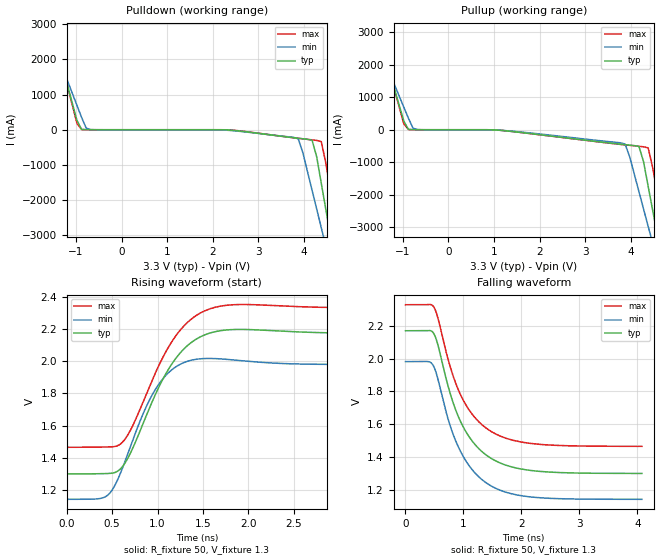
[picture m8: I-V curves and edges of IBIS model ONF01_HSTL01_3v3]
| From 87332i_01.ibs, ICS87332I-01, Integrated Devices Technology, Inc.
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[Model] ONF01_HSTL01_3v3
Model_type  Output_ECL
Polarity   Non-Inverting
Vmeas = 1.56
Rref = 50
Cref = 0
Vref = 1.3
|   typ   min   max
C_comp   4pF   3.6pF   4.4pF
|   typ   min   max
[Temperature Range]   25   -40   85
|   typ   min   max
[Voltage range]   3.3V   3.135V   3.465V
|   typ   min   max
[Pullup Reference]   3.3V   3.135V   3.465V
|   typ   min   max
[Pulldown Reference]   3.3V   3.135V   3.465V
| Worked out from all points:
|   rising waveform, R_fixture 50, V_fixture 1.3: 20-80 % time 436ps typ, 369ps min, 442ps max; typ from 1.3 V to 2.17 V
|   falling waveform, R_fixture 50, V_fixture 1.3: 20-80 % time 585ps typ, 578ps min, 582ps max; typ from 2.17 V to 1.3 V
| Open source, no load
|  Voltage   I(typ)   I(min)   I(max)
[Pulldown]
-3.3V     11.43A     8.569A     12.06A
-1.583V   3.173A     2.741A     3.273A
-1.482V   2.688A     2.399A     2.757A
-976.5mV  265.3mA    691.7mA    179.8mA
-875.5mV  9.277mA    351.3mA    5.817mA
-673.5mV  497.4uA    4.407mA    311.2uA
3.872V    -242.5mA   -258.2mA   -243.1mA
4.176V    -296.5mA   -1.72A     -288.3mA
4.378V    -1.523A    -2.788A    -338.2mA
4.58V     -3.033A    -3.855A    -1.761A
4.782V    -4.544A    -4.922A    -3.367A
6.6V      -18.28A    -14.6A     -17.98A
|  Voltage   I(typ)   I(min)   I(max)
[Pullup]
-3.3V     11.43A     8.569A     12.06A
-1.785V   4.144A     3.426A     4.306A
-1.583V   3.173A     2.741A     3.273A
-976.5mV  265.3mA    691.7mA    179.8mA
-875.5mV  9.277mA    351.3mA    5.817mA
-673.5mV  497.4uA    4.407mA    311.2uA
3.872V    -459.3mA   -442.5mA   -466.1mA
4.176V    -512mA     -1.904A    -509.8mA
4.378V    -1.738A    -2.972A    -558.7mA
4.58V     -3.247A    -4.039A    -1.98A
4.782V    -4.756A    -5.105A    -3.585A
6.6V      -18.37A    -14.72A    -18.06A
[Ramp]
|   typ   min   max
dV/dt_r   0.716/0.687n   0.698/0.591n   0.708/0.691n
dV/dt_f   0.696/0.94n   0.671/0.923n   0.691/0.935n
R_load =   50.0000
[Rising Waveform]
R_fixture = 50
V_fixture = 1.3   | VCC_typ - 2V
V_fixture_max = 1.465   | VCC_max - 2V
V_fixture_min = 1.135   | VCC_min - 2V
C_fixture = 0.0p
| Time   typ   min   max
0s        1.3V       1.142V     1.465V
427.6ps   1.302V     1.159V     1.467V
612.1ps   1.344V     1.334V     1.496V
731ps     1.465V     1.516V     1.605V
960.6ps   1.774V     1.81V      1.907V
1.121ns   1.95V      1.928V     2.087V
1.301ns   2.081V     1.993V     2.224V
1.522ns   2.163V     2.015V     2.312V
1.805ns   2.194V     2.008V     2.348V
3.867ns   2.17V      1.98V      2.328V
[Falling Waveform]
R_fixture = 50
V_fixture = 1.3   | VCC_typ - 2V
V_fixture_max = 1.465   | VCC_max - 2V
V_fixture_min = 1.135   | VCC_min - 2V
C_fixture = 0.0p
| Time   typ   min   max
0s        2.169V     1.981V     2.328V
395.7ps   2.171V     1.981V     2.329V
485.9ps   2.154V     1.953V     2.315V
559.7ps   2.083V     1.875V     2.247V
760.6ps   1.8V       1.602V     1.963V
941ps     1.623V     1.44V      1.786V
1.183ns   1.483V     1.309V     1.646V
1.482ns   1.391V     1.223V     1.555V
2.257ns   1.315V     1.154V     1.479V
4.077ns   1.3V       1.142V     1.465V
